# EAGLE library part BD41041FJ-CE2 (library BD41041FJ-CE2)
ROHM Semiconductor CAN Transceiver for Automotive Source: Datasheet
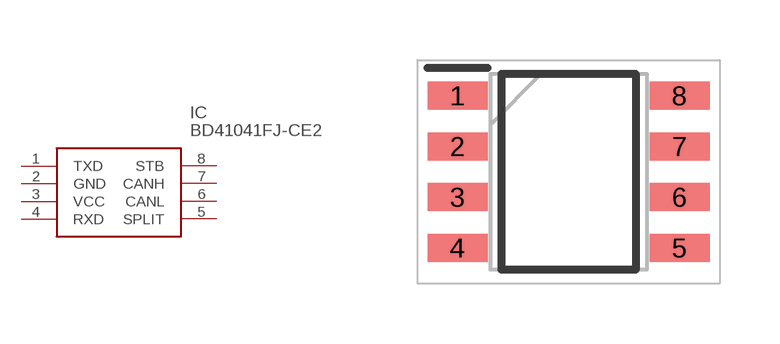
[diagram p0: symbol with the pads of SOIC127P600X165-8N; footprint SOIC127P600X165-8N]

Designator prefix IC

## BD41041FJ-CE2 (Description: ROHM Semiconductor CAN Transceiver for Automotive; Height: 1.65mm; Manufacturer_Name: ROHM Semiconductor; Manufacturer_Part_Number: BD41041FJ-CE2; Mouser_Part_Number: 755-BD41041FJ-CE2; Mouser_Price-Stock: https://www.mouser.co.uk/ProductDetail/ROHM-Semiconductor/BD41041FJ-CE2?qs=%252BEew9%252B0nqrCizAYMbF4Vxg%3D%3D)  [SOIC127P600X165-8N]
1  TXD
2  GND
3  VCC
4  RXD
5  SPLIT
6  CANL
7  CANH
8  STB

## Footprint SOIC127P600X165-8N (pad centres in mm)
SOP-J8
smd 1.5 x 0.7: 1 -2.775,1.905; 2 -2.775,0.635; 3 -2.775,-0.635; 4 -2.775,-1.905; 5 2.775,-1.905; 6 2.775,-0.635; 7 2.775,0.635; 8 2.775,1.905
